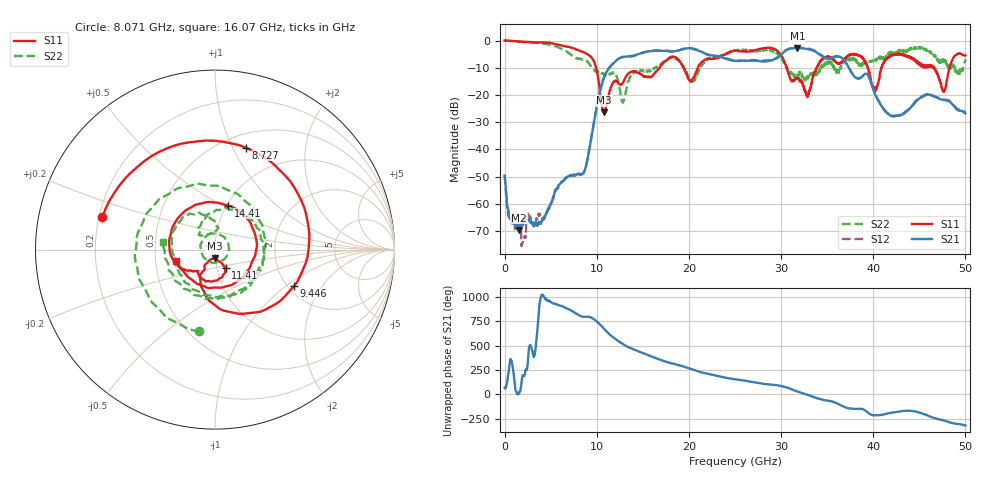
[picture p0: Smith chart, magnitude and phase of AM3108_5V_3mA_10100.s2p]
# Hz S DB R 50.0
!freq dBS11 angS11 dBS21 angS21 dBS12 angS12 dBS22 angS22
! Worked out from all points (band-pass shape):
!   1601 points, 10 MHz to 50 GHz, reference 50 ohm
!   highest |S21| = -2.75 dB at 31.78 GHz (marker M1); lowest = -69.5 dB at 1.572 GHz (marker M2)
!   |S21| within 3 dB of the highest: 13.93 GHz to 22.92 GHz (8.991 GHz wide, 48.8 % of centre); 29.86 GHz to 34.43 GHz (4.568 GHz wide, 14.2 % of centre)
!   lowest |S11| = -26.4 dB at 10.82 GHz (marker M3), VSWR 1.10, Z = 49.7 - j4.76 ohm
!   |S11| at or under -10 dB: 9.942 GHz to 16.83 GHz (6.886 GHz wide, 51.4 % of centre); 30.62 GHz to 33.85 GHz (3.229 GHz wide, 10 % of centre); 46.63 GHz to 48.28 GHz (1.656 GHz wide, 3.49 % of centre)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
!   |S22| runs from -22.9 to 0.0 dB; largest |S21 - S12| = 0.022
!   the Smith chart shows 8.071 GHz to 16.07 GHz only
!   S11 on the Smith chart (normalised r, x): 8.071 GHz: 0.21, +0.13; 8.727 GHz: 0.64, +1.13; 9.446 GHz: 2.15, -1.15; 11.41 GHz: 1.10, -0.23; 14.41 GHz: 1.02, +0.54; 16.07 GHz: 0.64, -0.08
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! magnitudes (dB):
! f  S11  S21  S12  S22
! 10 MHz  0.0  -49.6  -49.4  0.0
! 1.572 GHz  -0.4  -69.5  -69.3  -0.5
! 8.071 GHz  -3.7  -49.0  -49.2  -6.7
! 8.352 GHz  -4.0  -49.1  -49.2  -6.8
! 8.727 GHz  -4.5  -47.5  -47.3  -7.1
! 9.446 GHz  -6.3  -35.1  -34.9  -9.7
! 10.82 GHz  -26.4  -13.4  -13.3  -12.4
! 11.41 GHz  -18.4  -9.9  -9.7  -12.4
! 12.85 GHz  -15.4  -6.1  -6.0  -22.9
! 14.41 GHz  -11.8  -5.1  -5.1  -11.4
! 16.07 GHz  -12.9  -3.8  -3.6  -10.6
! 16.69 GHz  -10.5  -3.8  -3.6  -9.7
! 20.41 GHz  -14.1  -3.1  -2.9  -15.2
! 25 GHz  -3.7  -7.5  -7.3  -3.8
! 29.25 GHz  -3.0  -7.0  -6.8  -4.0
! 31.78 GHz  -14.1  -2.7  -2.6  -13.4
! 33.35 GHz  -15.5  -3.5  -3.3  -12.7
! 37.91 GHz  -5.0  -13.1  -12.9  -6.4
! 40.22 GHz  -18.6  -19.9  -19.6  -7.6
! 41.69 GHz  -6.1  -27.1  -27.1  -5.2
! 47.66 GHz  -18.9  -21.9  -21.7  -7.6
! 50 GHz  -5.5  -26.8  -26.6  -6.9
